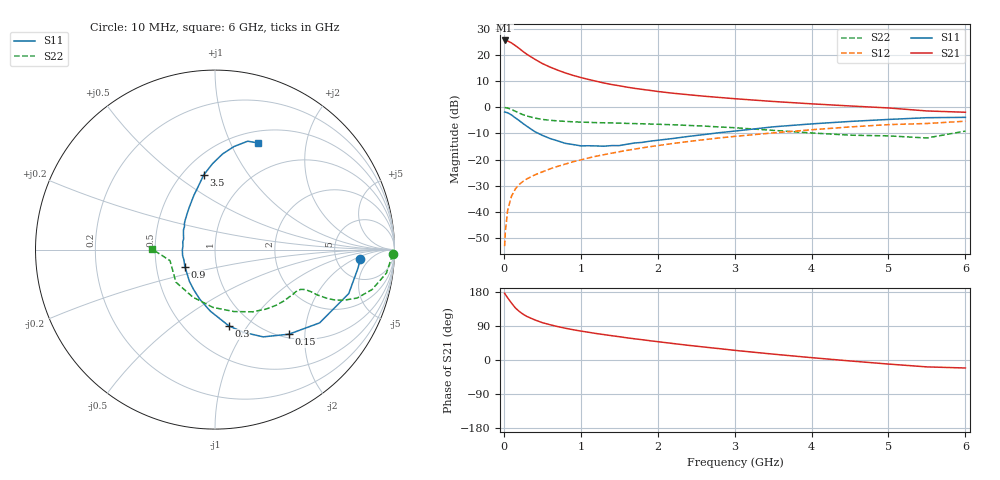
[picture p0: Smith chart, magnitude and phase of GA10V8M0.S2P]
! Infineon Technologies  Discrete & RF Semiconductors
! BF775
! Si NPN RF Bipolar Junction Transistor in SOT23
! VCE = 10 V  IC = 8 mA
! Common Emitter S-Parameters:  May  1996
# GHz  S  MA  R  50
!  f  S11  S21  S12  S22
! GHz  MAG  ANG  MAG  ANG  MAG  ANG  MAG  ANG
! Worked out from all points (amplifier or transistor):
!   36 points, 10 MHz to 6 GHz, reference 50 ohm
!   highest |S21| = 25.6 dB at 10 MHz (marker M1)
!   |S21| within 3 dB of that: start of sweep to 197.3 MHz
!   unconditionally stable (mu >= 1): 718.2 MHz to 2.82 GHz
!   at 250 MHz: K = 0.59, MSG = 24.8 dB, |S12| = -28.4 dB
!   at 1.4 GHz: K = 1.09, MAG = 11.3 dB, |S12| = -17.6 dB
!   at 6 GHz: K = 0.88, MSG = 1.7 dB, |S12| = -5.3 dB
!   S11 on the Smith chart (normalised r, x): 10 MHz: 8.67, -2.71; 150 MHz: 1.07, -1.66; 300 MHz: 0.79, -0.82; 900 MHz: 0.70, -0.14; 3.5 GHz: 0.63, +0.64; 6 GHz: 0.64, +1.28
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0.01  0.8101 -3.8  18.95 176.1  0.0022 91.5  0.9899 -1.5
0.02  0.8037 -7.3  18.8 172.9  0.0042 86.0  0.9819 -3.2
0.05  0.7844 -18.2  18.53 163.9  0.0108 79.2  0.964 -7.8
0.1  0.7117 -35.0  16.96 150.1  0.02 73.3  0.9028 -14.3
0.15  0.6256 -48.9  15.08 137.4  0.0274 68.2  0.837 -18.8
0.2  0.5554 -61.1  13.32 128.3  0.0334 64.8  0.7726 -21.4
0.25  0.4873 -71.0  11.64 120.9  0.0382 62.5  0.7199 -22.9
0.3  0.432 -79.7  10.3 114.9  0.0427 62.1  0.6803 -23.5
0.4  0.3431 -94.5  8.334 106.0  0.0506 62.0  0.6223 -23.9
0.5  0.2901 -106.8  6.866 98.6  0.058 62.5  0.5846 -23.7
0.6  0.2523 -118.2  5.87 93.1  0.0662 62.9  0.5632 -23.8
0.7  0.2272 -128.9  5.124 88.2  0.0741 63.3  0.5483 -24.0
0.9  0.1933 -150.3  4.067 79.9  0.0906 64.2  0.5265 -24.9
1.1  0.1834 -170.1  3.403 73.2  0.107 64.4  0.5139 -26.6
1.3  0.1795 173.6  2.913 67.1  0.1236 63.8  0.5039 -28.6
1.6  0.196 153.7  2.423 58.5  0.1495 62.3  0.4908 -32.5
2.2  0.2528 128.0  1.854 43.5  0.2028 58.4  0.4621 -41.9
2.8  0.3259 111.0  1.54 30.0  0.2583 53.3  0.4197 -53.8
3.5  0.4217 98.5  1.29 15.5  0.3229 45.8  0.3612 -72.9
4.5  0.5352 85.4  1.058 -2.5  0.4201 34.0  0.2922 -114.9
5.5  0.6309 73.2  0.849 -18.2  0.4889 18.9  0.2581 -166.2
6  0.641 67.8  0.802 -21.1  0.5405 14.7  0.3499 179.6
